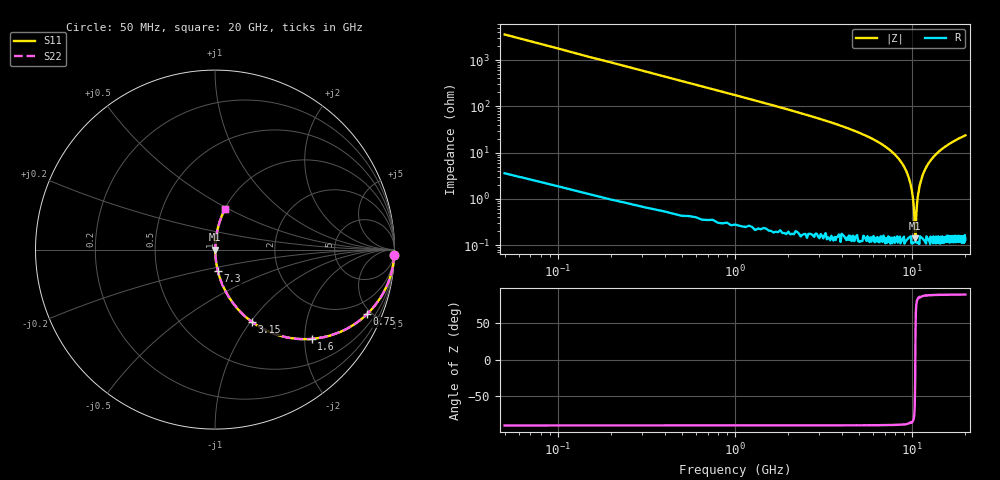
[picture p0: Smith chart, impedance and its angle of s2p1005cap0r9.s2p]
!	AVX	Thin	Film	Operation
!	Date:	March 2012
!	Description: Ultra-Miniature 01005 Size ACCU - P® Thin Film RF / Microwave Capacitor
!	Part Number:  C005YK0R9ABSTR
!	Serial	Measurements
# MHZ S MA R 50
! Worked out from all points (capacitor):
!   400 points, 50 MHz to 20 GHz, reference 50 ohm
!   read as one part in series: C = 900 fF near 150 MHz
!   lowest |Z| = 140 mohm at 10.4 GHz (marker M1)
!   series resonance near 10.42 GHz, so ESL is about 260 pH
!   S11 on the Smith chart (normalised r, x): 50 MHz: 0, -71; 750 MHz: 1.01, -4.69; 1.6 GHz: 1.00, -2.16; 3.15 GHz: 1.00, -1.02; 7.3 GHz: 1.00, -0.25; 20 GHz: 1.00, +0.47
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50  1 -1.6  0.028 88.3  0.028 88.3  1 -1.6
150  0.996 -4.8  0.085 85.1  0.085 85.1  0.996 -4.8
250  0.99 -8.1  0.14 81.9  0.14 81.9  0.99 -8.1
750  0.919 -23.1  0.392 66.8  0.392 66.8  0.919 -23.1
1600  0.733 -42.8  0.679 47.1  0.679 47.1  0.733 -42.8
3150  0.454 -62.8  0.89 27.0  0.89 27.0  0.454 -62.8
3400  0.421 -64.9  0.906 24.9  0.906 24.9  0.421 -64.9
6700  0.153 -80.7  0.987 8.8  0.987 8.8  0.153 -80.7
7300  0.122 -82.3  0.991 7.0  0.991 7.0  0.122 -82.3
9250  0.041 -85.8  0.998 2.3  0.998 2.3  0.041 -85.8
9750  0.023 -85.4  0.998 1.3  0.998 1.3  0.023 -85.4
10050  0.012 -83.2  0.999 0.7  0.999 0.7  0.012 -83.2
10250  0.005865 -76.7  0.999 0.3  0.999 0.3  0.005865 -76.7
10400  0.001537 -31.0  0.999 0.0  0.999 0.0  0.001537 -31.0
10450  0.001559 32.2  0.999 -0.0  0.999 -0.0  0.001559 32.2
10550  0.004268 71.8  0.999 -0.2  0.999 -0.2  0.004268 71.8
10750  0.011 82.2  0.999 -0.6  0.999 -0.6  0.011 82.2
11150  0.023 85.4  0.998 -1.3  0.998 -1.3  0.023 85.4
12100  0.051 85.6  0.997 -2.9  0.997 -2.9  0.051 85.6
13350  0.084 84.3  0.995 -4.8  0.995 -4.8  0.084 84.3
16700  0.163 80.1  0.985 -9.4  0.985 -9.4  0.163 80.1
20000  0.23 76.3  0.972 -13.3  0.972 -13.3  0.23 76.3
